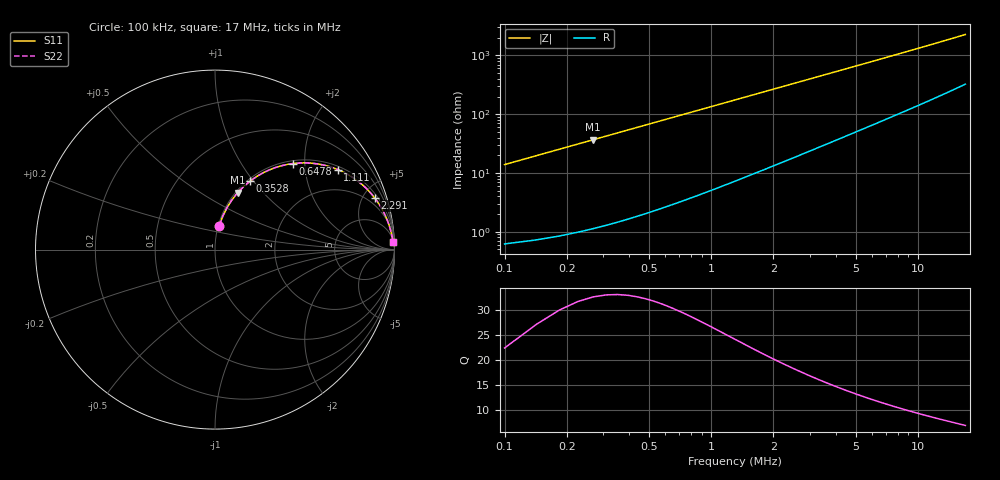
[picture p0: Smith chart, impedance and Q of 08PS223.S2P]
! Coilcraft 0805PS-223 Power Chip Inductor
! 5 February 2003
# MHZ S MA R 50
!Freq  MagS11  AngS11  MagS21  AngS21  MagS12  AngS12  MagS22  AngS22
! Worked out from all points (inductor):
!   403 points, 100 kHz to 17 MHz, reference 50 ohm
!   read as one part in series: L = 21.8 uH near 184.3 kHz
!   highest Q = 32.6 at 268.6 kHz (marker M1), where L = 21.8 uH
!   S11 on the Smith chart (normalised r, x): 100 kHz: 1.01, +0.28; 352.8 kHz: 1.03, +0.96; 647.8 kHz: 1.06, +1.75; 1.111 MHz: 1.12, +2.98; 2.291 MHz: 1.32, +6.08; 17 MHz: 7, +45
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0.1  0.1365 79.6  0.9846 -7.8  0.9846 -7.8  0.1365 79.6
0.14214  0.1911 76.9  0.9746 -11.0  0.9746 -11.0  0.1911 76.9
0.18428  0.2436 74.0  0.9618 -14.1  0.9618 -14.1  0.2436 74.0
0.22642  0.2938 71.1  0.9467 -17.1  0.9467 -17.1  0.2938 71.1
0.26856  0.3413 68.3  0.9295 -19.9  0.9295 -19.9  0.3413 68.3
0.35284  0.4282 62.9  0.8908 -25.3  0.8908 -25.3  0.4282 62.9
0.47926  0.5375 55.7  0.8268 -32.5  0.8268 -32.5  0.5375 55.7
0.64782  0.6481 47.7  0.7405 -40.4  0.7405 -40.4  0.6481 47.7
0.85852  0.7431 40.0  0.6432 -48.0  0.6432 -48.0  0.7431 40.0
1.11136  0.8158 33.2  0.5474 -54.6  0.5474 -54.6  0.8158 33.2
1.3642  0.8617 28.2  0.4724 -59.4  0.4724 -59.4  0.8617 28.2
1.61704  0.892 24.4  0.4135 -63.0  0.4135 -63.0  0.892 24.4
1.91202  0.9157 21.1  0.3598 -66.2  0.3598 -66.2  0.9157 21.1
2.29128  0.9356 17.9  0.3075 -69.1  0.3075 -69.1  0.9356 17.9
2.92338  0.9547 14.3  0.2467 -72.4  0.2467 -72.4  0.9547 14.3
4.18758  0.9723 10.1  0.1761 -75.9  0.1761 -75.9  0.9723 10.1
5.74676  0.9811 7.4  0.1299 -77.9  0.1299 -77.9  0.9811 7.4
7.0531  0.9849 6.1  0.1063 -78.8  0.1063 -78.8  0.9849 6.1
8.57014  0.9876 5.0  0.08773 -79.4  0.08773 -79.4  0.9876 5.0
11.39352  0.9903 3.8  0.06597 -79.7  0.06597 -79.7  0.9903 3.8
14.2169  0.9919 3.0  0.05261 -79.6  0.05261 -79.6  0.9919 3.0
17  0.9928 2.5  0.04363 -79.3  0.04363 -79.3  0.9928 2.5
